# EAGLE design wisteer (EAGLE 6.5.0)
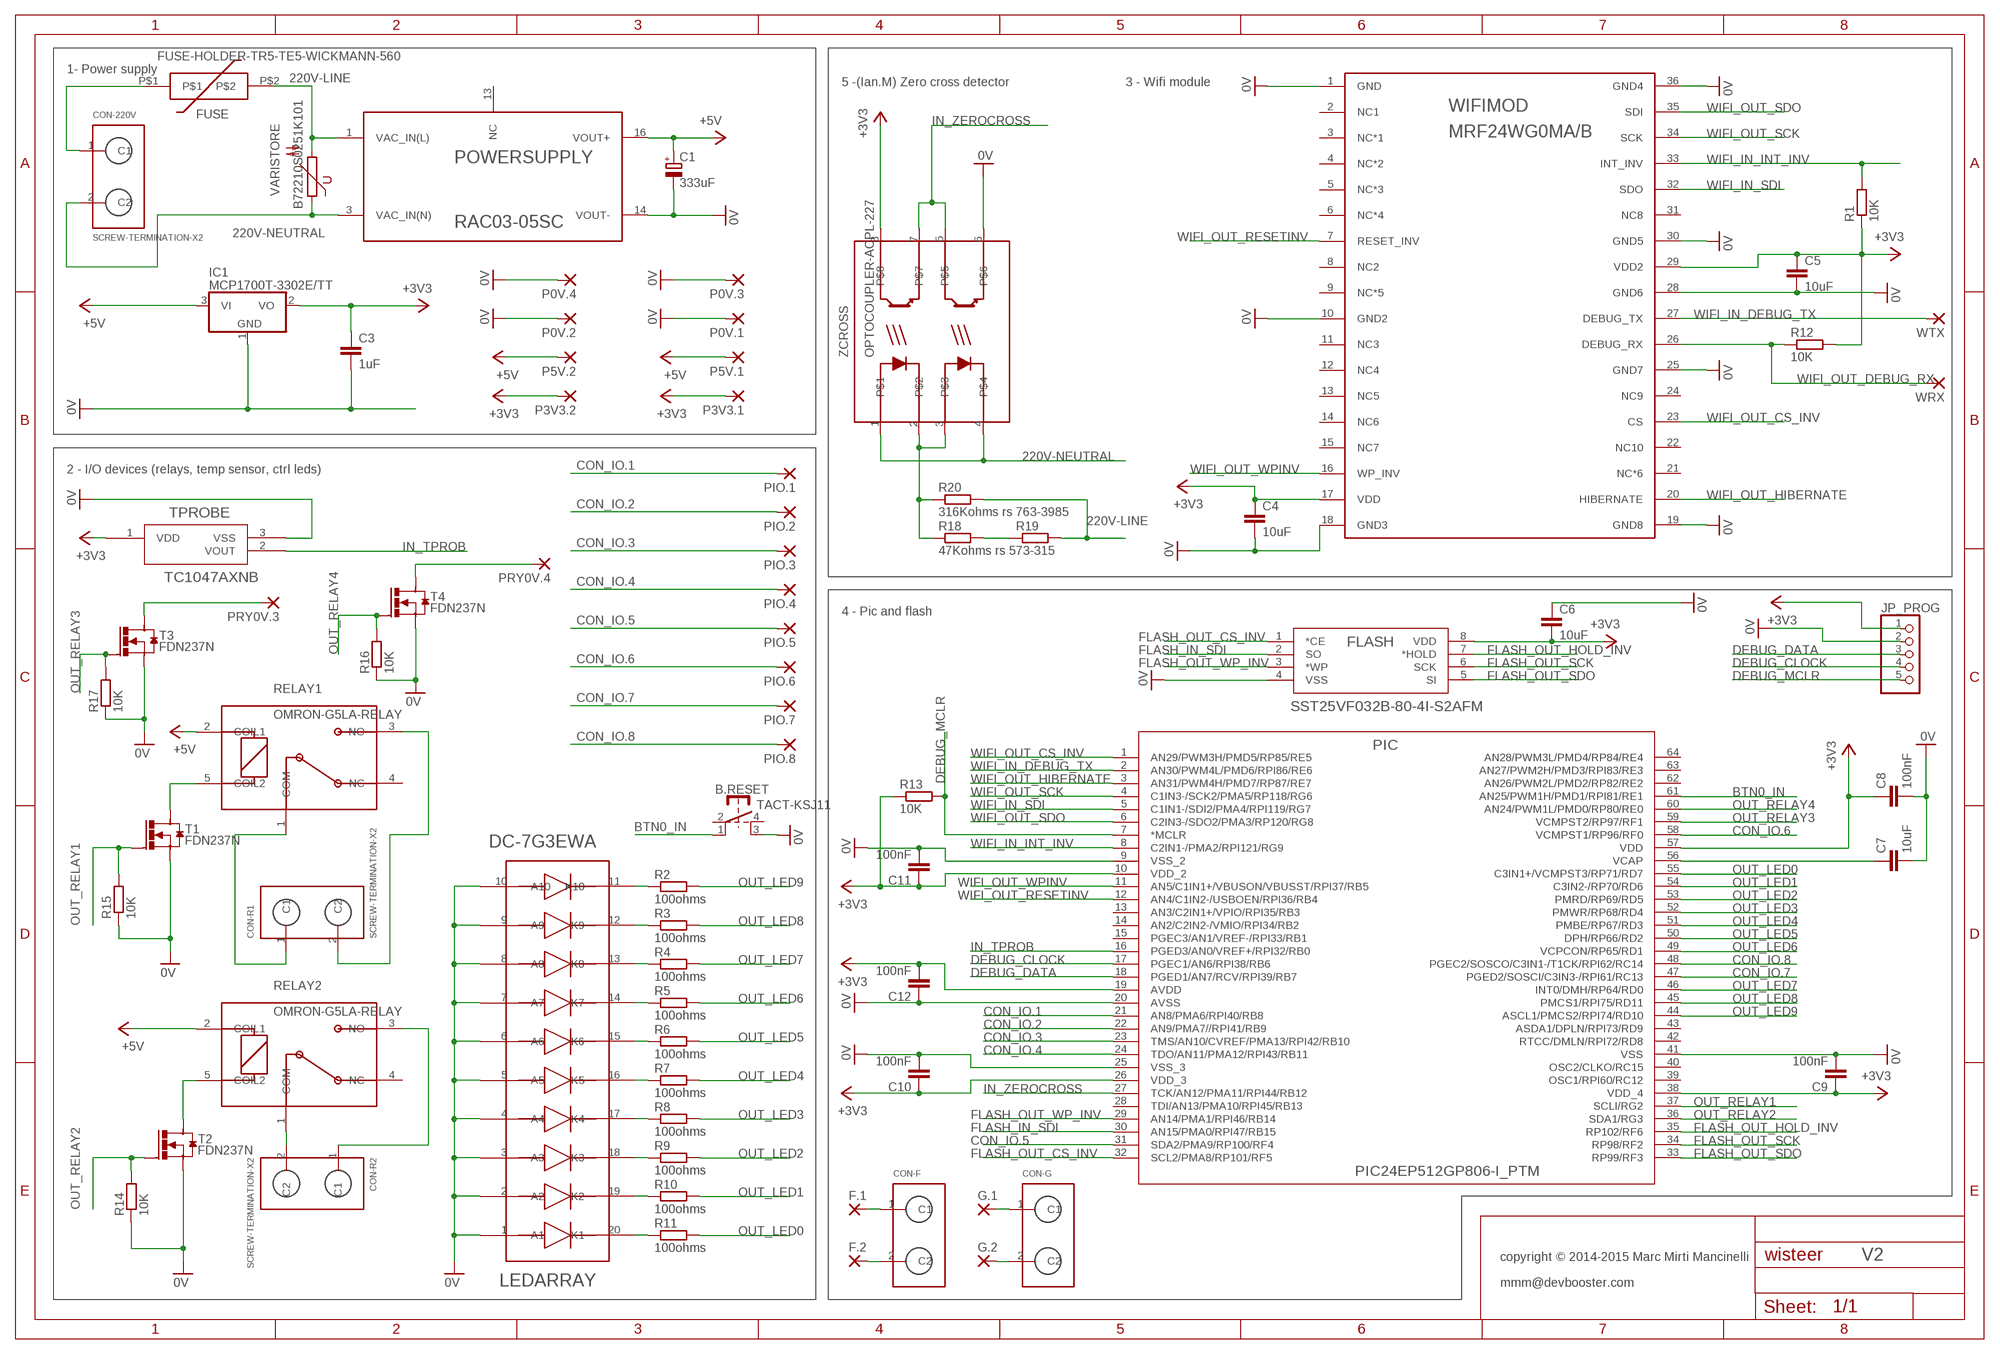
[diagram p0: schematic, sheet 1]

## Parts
B.RESET  TACT-KSJ11  [TACT-KSJ11]
C1  333uF  CPOL-EUTT5D10  [TT5D10]
C3  1uF  C-EUC0805  [C0805]
C4  10uF  C-EUC1210  [C1210]
C5  10uF  C-EUC1210  [C1210]
C6  10uF  C-EUC1210  [C1210]
C7  10uF  C-EUC1210  [C1210]
C8  100nF  C-EUC0603  [C0603]
C9  100nF  C-EUC0603  [C0603]
C10  100nF  C-EUC0603  [C0603]
C11  100nF  C-EUC0603  [C0603]
C12  100nF  C-EUC0603  [C0603]
CON-220V  SCREW-TERMINATION-X2  [PM5.08-2-90]
CON-F  SCREW-TERMINATION-X22.54  [MPT0.5-2-2.54]
CON-G  SCREW-TERMINATION-X22.54  [MPT0.5-2-2.54]
CON-R1  SCREW-TERMINATION-X2  [PM5.08-2-90]
CON-R2  SCREW-TERMINATION-X2  [PM5.08-2-90]
F.1  1,6/0,8  [1,6/0,8]
F.2  1,6/0,8  [1,6/0,8]
FLASH  SST25VF032B-80-4I-S2AFM  [SOIC8_S2A_SST-M]
FUSE  FUSE-HOLDER-TR5-TE5-WICKMANN-560  [FUSE-HOLDER-TR5-TE5-WICKMANN-560]
G.1  1,6/0,8  [1,6/0,8]
G.2  1,6/0,8  [1,6/0,8]
IC1  MCP1700T-3302E/TT  MCP1703CB  [SOT23]
JP_PROG  PINHD-1X5  [1X05]
LEDARRAY  DC-7G3EWA  10-SEGMENT-LED-ARRAY  [10-SEG-LED-DC-7G3EWA]
P0V.1  1,6/0,8  [1,6/0,8]
P0V.2  1,6/0,8  [1,6/0,8]
P0V.3  1,6/0,8  [1,6/0,8]
P0V.4  1,6/0,8  [1,6/0,8]
P3V3.1  1,6/0,8  [1,6/0,8]
P3V3.2  1,6/0,8  [1,6/0,8]
P5V.1  1,6/0,8  [1,6/0,8]
P5V.2  1,6/0,8  [1,6/0,8]
PIC  PIC24EP512GP806-I_PTM  [QFP64-10X10MC-M]
PIO.1  1,6/0,8  [1,6/0,8]
PIO.2  1,6/0,8  [1,6/0,8]
PIO.3  1,6/0,8  [1,6/0,8]
PIO.4  1,6/0,8  [1,6/0,8]
PIO.5  1,6/0,8  [1,6/0,8]
PIO.6  1,6/0,8  [1,6/0,8]
PIO.7  1,6/0,8  [1,6/0,8]
PIO.8  1,6/0,8  [1,6/0,8]
POWERSUPPLY  RAC03-05SC  [RAC03-05SC]
PRY0V.3  1,6/0,8  [1,6/0,8]
PRY0V.4  1,6/0,8  [1,6/0,8]
R1  10K  R-EU_R0603  [R0603]
R2  100ohms  R-EU_R0603  [R0603]
R3  100ohms  R-EU_R0603  [R0603]
R4  100ohms  R-EU_R0603  [R0603]
R5  100ohms  R-EU_R0603  [R0603]
R6  100ohms  R-EU_R0603  [R0603]
R7  100ohms  R-EU_R0603  [R0603]
R8  100ohms  R-EU_R0603  [R0603]
R9  100ohms  R-EU_R0603  [R0603]
R10  100ohms  R-EU_R0603  [R0603]
R11  100ohms  R-EU_R0603  [R0603]
R12  10K  R-EU_R0603  [R0603]
R13  10K  R-EU_R0603  [R0603]
R14  10K  R-EU_R0603  [R0603]
R15  10K  R-EU_R0603  [R0603]
R16  10K  R-EU_R0603  [R0603]
R17  10K  R-EU_R0603  [R0603]
R18  47Kohms rs 573-315  R-EU_R1206W  [R1206W]
R19  47Kohms rs 573-315  R-EU_R1206W  [R1206W]
R20  316Kohms rs 763-3985  R-EU_R0805W  [R0805W]
RELAY1  OMRON-G5LA-RELAY  [OMRON-G5LA-RELAY]
RELAY2  OMRON-G5LA-RELAY  [OMRON-G5LA-RELAY]
T1  FDN237N  [SUPERSOT-3]
T2  FDN237N  [SUPERSOT-3]
T3  FDN237N  [SUPERSOT-3]
T4  FDN237N  [SUPERSOT-3]
TPROBE  TC1047AXNB  [SOT-23_MC]
VARISTORE  B72210S0251K101  S10K250  [S10K250]
WIFIMOD  MRF24WG0MA/B  MRF24WG0MA  [MRF24WG0MA]
WRX  1,6/0,8  [1,6/0,8]
WTX  1,6/0,8  [1,6/0,8]
ZCROSS  OPTOCOUPLER-ACPL-227  [SOIC8_S2A_SST-M]

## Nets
0V: B.RESET.3(S1) C1.- C3.2 C4.2 C5.2 C6.1 C7.2 C8.2 C9.2 C10.2 C11.2 C12.1 FLASH.4(VSS) IC1.1(GND) JP_PROG.2 LEDARRAY.1(A1) LEDARRAY.2(A2) LEDARRAY.3(A3) LEDARRAY.4(A4) LEDARRAY.5(A5) LEDARRAY.6(A6) LEDARRAY.7(A7) LEDARRAY.8(A8) LEDARRAY.9(A9) LEDARRAY.10(A10) P0V.1.1(P) P0V.2.1(P) P0V.3.1(P) P0V.4.1(P) PIC.9(VSS_2) PIC.20(AVSS) PIC.25(VSS_3) PIC.41(VSS) POWERSUPPLY.14(VOUT-) R14.1 R15.1 R16.1 R17.1 T1.2(S) T2.2(S) T3.2(S) T4.2(S) TPROBE.3(VSS) WIFIMOD.1(GND) WIFIMOD.10(GND2) WIFIMOD.18(GND3) WIFIMOD.19(GND8) WIFIMOD.25(GND7) WIFIMOD.28(GND6) WIFIMOD.30(GND5) WIFIMOD.36(GND4) ZCROSS.6
220V-LINE [220VPOWER]: FUSE.P$2 POWERSUPPLY.1(VAC_IN(L)) R19.2 R20.2 VARISTORE.2
220V-NEUTRAL [220VPOWER]: CON-220V.2(C2) POWERSUPPLY.3(VAC_IN(N)) VARISTORE.1 ZCROSS.1 ZCROSS.4
+3V3: C3.1 C4.1 C5.1 C6.2 C8.1 C9.1 C10.1 C11.1 C12.2 FLASH.8(VDD) IC1.2(VO) JP_PROG.1 P3V3.1.1(P) P3V3.2.1(P) PIC.10(VDD_2) PIC.19(AVDD) PIC.26(VDD_3) PIC.38(VDD_4) PIC.57(VDD) R1.1 R12.2 R13.1 TPROBE.1(VDD) WIFIMOD.17(VDD) WIFIMOD.29(VDD2) ZCROSS.8
+5V: C1.+ IC1.3(VI) P5V.1.1(P) P5V.2.1(P) POWERSUPPLY.16(VOUT+) RELAY1.2(COIL1) RELAY2.2(COIL1)
BTN0_IN: B.RESET.1 PIC.61(AN25/PWM1H/PMD1/RPI81/RE1)
CON_IO.1: PIC.21(AN8/PMA6/RPI40/RB8) PIO.1.1(P)
CON_IO.2: PIC.22(AN9/PMA7//RPI41/RB9) PIO.2.1(P)
CON_IO.3: PIC.23(TMS/AN10/CVREF/PMA13/RPI42/RB10) PIO.3.1(P)
CON_IO.4: PIC.24(TDO/AN11/PMA12/RPI43/RB11) PIO.4.1(P)
CON_IO.5: PIC.31(SDA2/PMA9/RP100/RF4) PIO.5.1(P)
CON_IO.6: PIC.58(VCMPST1/RP96/RF0) PIO.6.1(P)
CON_IO.7: PIC.47(PGED2/SOSCI/C3IN3-/RPI61/RC13) PIO.7.1(P)
CON_IO.8: PIC.48(PGEC2/SOSCO/C3IN1-/T1CK/RPI62/RC14) PIO.8.1(P)
DEBUG_CLOCK: JP_PROG.4 PIC.17(PGEC1/AN6/RPI38/RB6)
DEBUG_DATA: JP_PROG.3 PIC.18(PGED1/AN7/RCV/RPI39/RB7)
DEBUG_MCLR: JP_PROG.5 PIC.7(*MCLR) R13.2
FLASH_IN_SDI: FLASH.2(SO) PIC.30(AN15/PMA0/RPI47/RB15)
FLASH_OUT_CS_INV: FLASH.1(*CE) PIC.32(SCL2/PMA8/RP101/RF5)
FLASH_OUT_HOLD_INV: FLASH.7(*HOLD) PIC.35(RP102/RF6)
FLASH_OUT_SCK: FLASH.6(SCK) PIC.34(RP98/RF2)
FLASH_OUT_SDO: FLASH.5(SI) PIC.33(RP99/RF3)
FLASH_OUT_WP_INV: FLASH.3(*WP) PIC.29(AN14/PMA1/RPI46/RB14)
IN_TPROB: PIC.16(PGED3/AN0/VREF+/RPI32/RB0) TPROBE.2(VOUT)
IN_ZEROCROSS: PIC.27(TCK/AN12/PMA11/RPI44/RB12) ZCROSS.5 ZCROSS.7
N$2: R18.1 R20.1 ZCROSS.2 ZCROSS.3
N$3 [220VRELAY]: CON-R2.2(C2) RELAY2.1(COM)
N$4 [220VRELAY]: CON-R2.1(C1) RELAY2.3(NO)
N$5 [220VRELAY]: CON-R1.1(C1) RELAY1.1(COM)
N$6 [220VRELAY]: CON-R1.2(C2) RELAY1.3(NO)
N$7: LEDARRAY.11(K10) R2.1
N$8: RELAY2.5(COIL2) T2.3(D)
N$9: LEDARRAY.12(K9) R3.1
N$10: LEDARRAY.13(K8) R4.1
N$11: LEDARRAY.14(K7) R5.1
N$12: RELAY1.5(COIL2) T1.3(D)
N$13: LEDARRAY.15(K6) R6.1
N$14: LEDARRAY.16(K5) R7.1
N$15: LEDARRAY.17(K4) R8.1
N$16: LEDARRAY.18(K3) R9.1
N$17: LEDARRAY.19(K2) R10.1
N$18: LEDARRAY.20(K1) R11.1
N$19: C7.1 PIC.56(VCAP)
N$20 [220VPOWER]: CON-220V.1(C1) FUSE.P$1
N$21: CON-F.1(C1) F.1.1(P)
N$22: CON-F.2(C2) F.2.1(P)
N$23: CON-G.1(C1) G.1.1(P)
N$24: CON-G.2(C2) G.2.1(P)
N$25: R18.2 R19.1
OUT_LED0: PIC.55(C3IN1+/VCMPST3/RP71/RD7) R11.2
OUT_LED1: PIC.54(C3IN2-/RP70/RD6) R10.2
OUT_LED2: PIC.53(PMRD/RP69/RD5) R9.2
OUT_LED3: PIC.52(PMWR/RP68/RD4) R8.2
OUT_LED4: PIC.51(PMBE/RP67/RD3) R7.2
OUT_LED5: PIC.50(DPH/RP66/RD2) R6.2
OUT_LED6: PIC.49(VCPCON/RP65/RD1) R5.2
OUT_LED7: PIC.46(INT0/DMH/RP64/RD0) R4.2
OUT_LED8: PIC.45(PMCS1/RPI75/RD11) R3.2
OUT_LED9: PIC.44(ASCL1/PMCS2/RPI74/RD10) R2.2
OUT_RELAY1: PIC.37(SCLI/RG2) R15.2 T1.1(G)
OUT_RELAY2: PIC.36(SDA1/RG3) R14.2 T2.1(G)
OUT_RELAY3: PIC.59(VCMPST2/RP97/RF1) R17.2 T3.1(G)
OUT_RELAY4: PIC.60(AN24/PWM1L/PMD0/RP80/RE0) R16.2 T4.1(G)
SRY0V.2: PRY0V.4.1(P) T4.3(D)
SRY0V.3: PRY0V.3.1(P) T3.3(D)
WIFI_IN_DEBUG_TX: PIC.2(AN30/PWM4L/PMD6/RPI86/RE6) WIFIMOD.27(DEBUG_TX) WTX.1(P)
WIFI_IN_INT_INV: PIC.8(C2IN1-/PMA2/RPI121/RG9) R1.2 WIFIMOD.33(INT_INV)
WIFI_IN_SDI: PIC.5(C1IN1-/SDI2/PMA4/RPI119/RG7) WIFIMOD.32(SDO)
WIFI_OUT_CS_INV: PIC.1(AN29/PWM3H/PMD5/RP85/RE5) WIFIMOD.23(CS)
WIFI_OUT_DEBUG_RX: R12.1 WIFIMOD.26(DEBUG_RX) WRX.1(P)
WIFI_OUT_HIBERNATE: PIC.3(AN31/PWM4H/PMD7/RP87/RE7) WIFIMOD.20(HIBERNATE)
WIFI_OUT_RESETINV: PIC.12(AN4/C1IN2-/USBOEN/RPI36/RB4) WIFIMOD.7(RESET_INV)
WIFI_OUT_SCK: PIC.4(C1IN3-/SCK2/PMA5/RP118/RG6) WIFIMOD.34(SCK)
WIFI_OUT_SDO: PIC.6(C2IN3-/SDO2/PMA3/RP120/RG8) WIFIMOD.35(SDI)
WIFI_OUT_WPINV: PIC.11(AN5/C1IN1+/VBUSON/VBUSST/RPI37/RB5) WIFIMOD.16(WP_INV)
Unconnected: B.RESET.2(P) B.RESET.4(S) PIC.13(AN3/C2IN1+/VPIO/RPI35/RB3) PIC.14(AN2/C2IN2-/VMIO/RPI34/RB2) PIC.15(PGEC3/AN1/VREF-/RPI33/RB1) PIC.28(TDI/AN13/PMA10/RPI45/RB13) PIC.39(OSC1/RPI60/RC12) PIC.40(OSC2/CLKO/RC15) PIC.42(RTCC/DMLN/RPI72/RD8) PIC.43(ASDA1/DPLN/RPI73/RD9) PIC.62(AN26/PWM2L/PMD2/RP82/RE2) PIC.63(AN27/PWM2H/PMD3/RPI83/RE3) PIC.64(AN28/PWM3L/PMD4/RP84/RE4) POWERSUPPLY.13(NC) RELAY1.4(NC) RELAY2.4(NC) WIFIMOD.2(NC1) WIFIMOD.3(NC*1) WIFIMOD.4(NC*2) WIFIMOD.5(NC*3) WIFIMOD.6(NC*4) WIFIMOD.8(NC2) WIFIMOD.9(NC*5) WIFIMOD.11(NC3) WIFIMOD.12(NC4) WIFIMOD.13(NC5) WIFIMOD.14(NC6) WIFIMOD.15(NC7) WIFIMOD.21(NC*6) WIFIMOD.22(NC10) WIFIMOD.24(NC9) WIFIMOD.31(NC8)

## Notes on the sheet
- 1- Power supply
- 5 -(Ian.M) Zero cross detector | 3 - Wifi module
- 2 - I/O devices (relays, temp sensor, ctrl leds)
- 4 - Pic and flash
- copyright © 2014-2015 Marc Mirti Mancinelli | V2
- mmm@devbooster.com

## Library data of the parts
B.RESET = mmm:TACT-KSJ11: KSJ11: KSJ Series Spherical Actuator Tact Switches Doc: http://www.madvapes.com/assets/images/ksj11.pdf madvapes ref: Item Id: 10117
C1 = rcl:CPOL-EU: POLARIZED CAPACITOR, European symbol
C3-C12 = rcl:C-EU: CAPACITOR, European symbol
CON-220V CON-F CON-G CON-R1 CON-R2 = comps for wipee:SCREW-TERMINATION-X2: PM5.08-2-90 5.08mm spacement
F.1 F.2 G.1 G.2 P0V.1-P0V.4 P3V3.1 P3V3.2 P5V.1 P5V.2 PIO.1-PIO.8 PRY0V.3 PRY0V.4 WRX WTX = wirepad:1,6/0,8: THROUGH-HOLE PAD
FLASH = comps for wipee:SST25VF032B-80-4I-S2AF: SST25VF032B-50-4I-S2AF: Flash memory (32Mbits) http://ww1.microchip.com/downloads/en/DeviceDoc/25071A.pdf
FUSE = comps for wipee:FUSE-HOLDER-TR5-TE5-WICKMANN-560: TR5/TE5 Fuse
IC1 = linear:MCP1703: 250 mA, 16V, Low Quiescent Current LDO Regulator Source: http://ww1.microchip.com/downloads/en/DeviceDoc/22049b.pdf
JP_PROG = pinhead:PINHD-1X5: PIN HEADER
LEDARRAY = comps for wipee:10-SEGMENT-LED-ARRAY: DC-7G3EWA :led array (rs 247-3107) http://radiospares-fr.rs-online.com/web/p/afficheurs-led/2473107/
PIC = comps for wipee:PIC24EP512GP806-I_PT: PIC24EP512GP806-I/PT: Pic with 512KB rom, 50KB ram, 60/70Mhz, 64 pins http://ww1.microchip.com/downloads/en/DeviceDoc/70616g.pdf
POWERSUPPLY = comps for wipee:RAC03-05SC: RAC03-05SC Power supply http://radiospares-fr.rs-online.com/web/p/alimentations-a-decoupage-integrables/7398339/
R1-R20 = rcl:R-EU_: RESISTOR, European symbol
RELAY1 RELAY2 = comps for wipee:OMRON-G5LA-RELAY: OMRON-G5LA-RELAY 5v, SPDT, 0.36W http://radiospares-fr.rs-online.com/web/p/relais-sans-accrochage/6839138/
T1-T4 = mmm:FDN237N: MOSFET CANAL N FDN237N Fairchild semiconductors http://docs-europe.electrocomponents.com/webdocs/0d23/0900766b80d23106.pdf
TPROBE = microchip tfrog:TC1047AXNB: Temperature sensor (TC1047AVNBTR) TC1047A can accurately measure temperature from -40C to +125C. For the TC1047A, the output voltage range is typically 100mV at -40C, 500mV at 0C, 750mV at +25C, and 1.75V at +125C. A 10mV/°C http://www.microchip.com/wwwproducts/Devices.aspx?dDocName=en010753#1
VARISTORE = varistor:S10K250: VARISTOR
WIFIMOD = comps for wipee:MRF24WG0MA: MRF24WG0MA Wifi module G/B with integrated antenna. http://ww1.microchip.com/downloads/en/DeviceDoc/70686B.pdf
ZCROSS = comps for wipee:OPTOCOUPLER-ACPL-227: Avago ACPL-227-50CE DC Input, Transistor Output Dual Optocoupler, SMT SOIC 8 2 channels, 50ma, 1.4v, delays 2us-3us Doc: http://docs-europe.electrocomponents.com/webdocs/0db7/0900766b80db7ce4.pdf Ref RS: 693-6797

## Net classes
0 default: clearance 0.205 mm
1 220VPOWER: clearance 0.5 mm
2 220VRELAY: clearance 0.5 mm

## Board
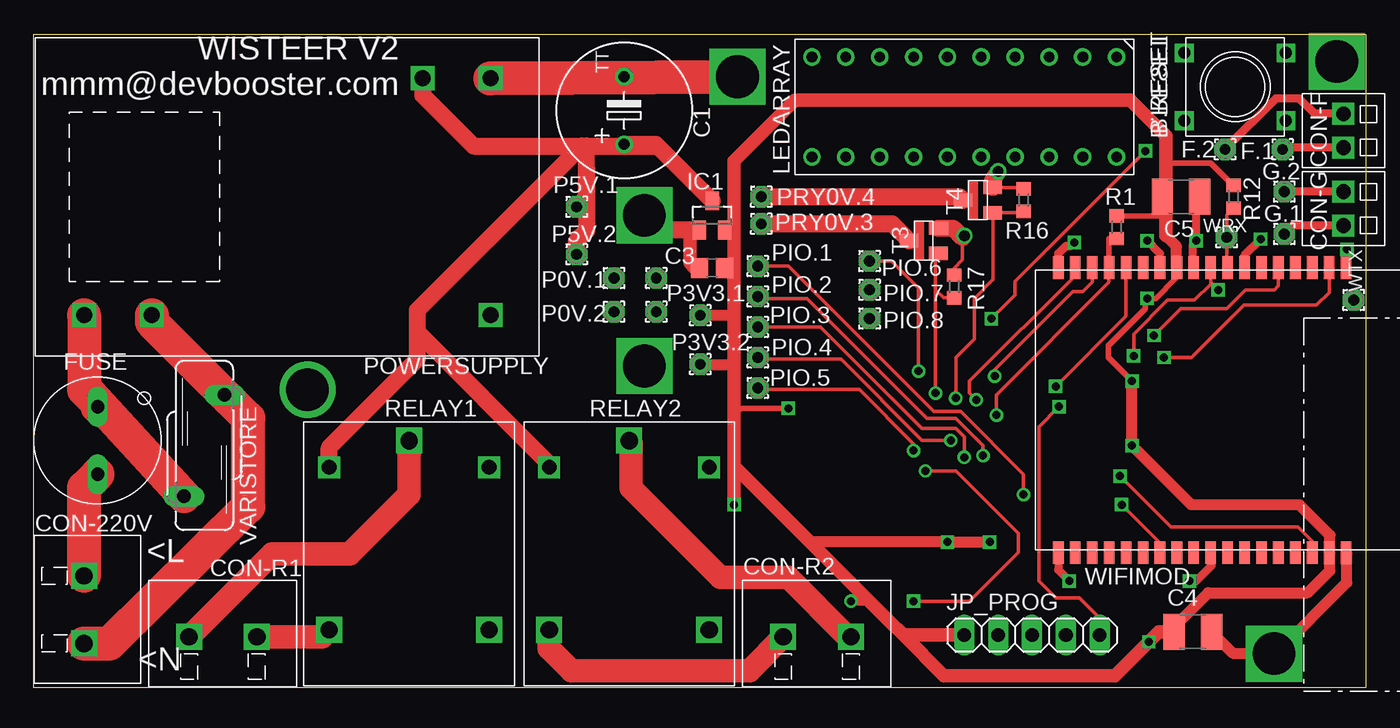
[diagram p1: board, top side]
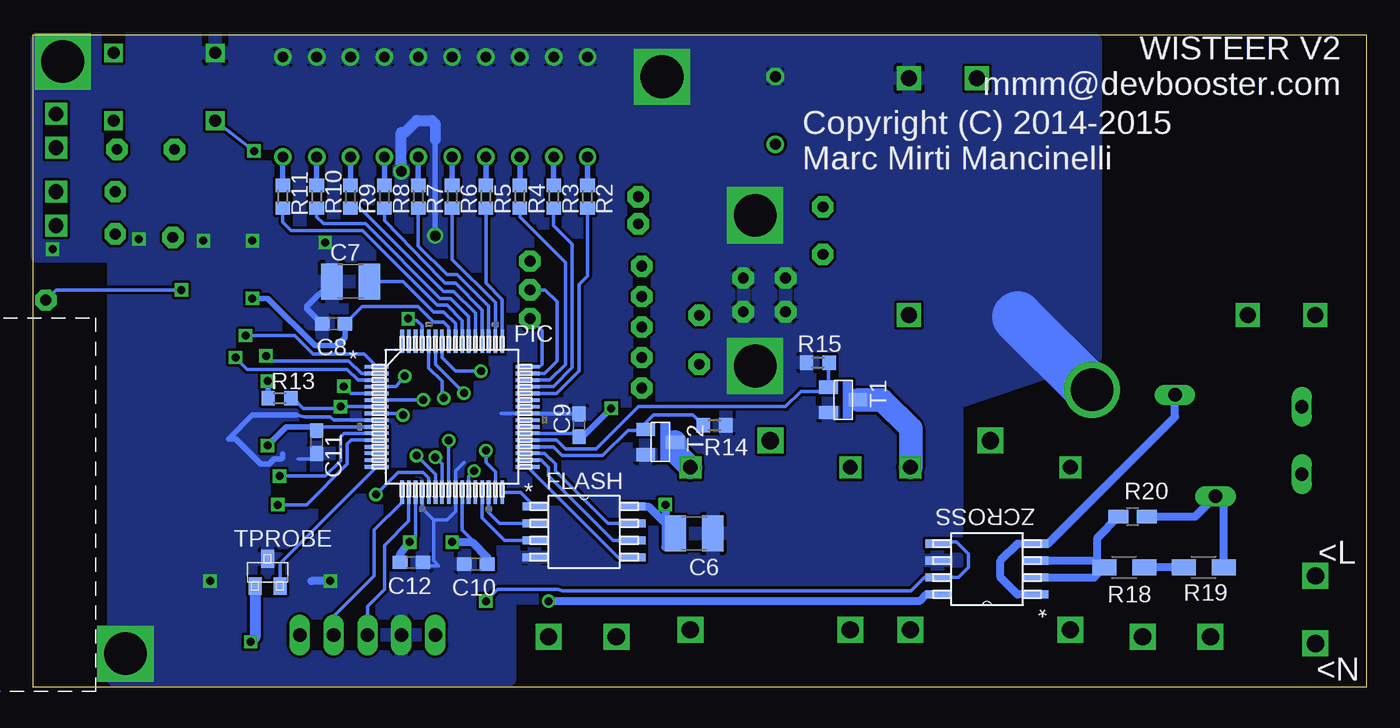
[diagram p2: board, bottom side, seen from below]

Size 100 x 49 mm. Coordinates in mm from the lower left corner, seen from the top.
Outline: 0,0 100,0 100,49 0,49 0,0
Copper layers (1*16): Top 0.035mm / dielectric 1.5mm / Bottom 0.035mm
Design rules "default *": minimum track width 10mil, minimum drill 16mil, track to track 8mil, track to pad 8mil, pad to pad 8mil, via to via 8mil, smd to smd 8mil, copper to edge 0mil, drill to drill 8mil, minimum pad ring 10mil, minimum via ring 8mil, stop-mask expansion 4mil, vias tented up to drill 0mil, thermal gap 10mil

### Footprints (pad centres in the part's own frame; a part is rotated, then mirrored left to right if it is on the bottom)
TACT-KSJ11 = drill 0.9 square: 1 -3.81,-2.54; 2 3.81,-2.54; 3 -3.81,2.54; 4 3.81,2.54
TT5D10 = drill 0.813: + -2.54,0 | drill 0.813 octagon: - 2.54,0
C0805 = smd 1.3 x 1.5: 1 -0.95,0; 2 0.95,0
C1210 = smd 1.6 x 2.7: 1 -1.4,0; 2 1.4,0
C0603 = smd 1.1 x 1: 1 -0.85,0; 2 0.85,0
PM5.08-2-90 = drill 1.3 square: 1 -2.54,0; 2 2.54,0
MPT0.5-2-2.54 = drill 1.1 square: 1 -1.27,0; 2 1.27,0
1,6/0,8 = drill 0.813 pad 1.6 octagon: 1 0,0
SOIC8_S2A_SST-M = smd 1.829 x 0.61: 1 -3.708,1.905; 2 -3.708,0.635; 3 -3.708,-0.635; 4 -3.708,-1.905; 5 3.708,-1.905; 6 3.708,-0.635; 7 3.708,0.635; 8 3.708,1.905
FUSE-HOLDER-TR5-TE5-WICKMANN-560 = drill 1 long: P$1 -2.54,0; P$2 2.54,0
SOT23 = smd 1 x 1.4: 1 -0.95,-1.1; 2 0.95,-1.1; 3 0,1.1
1X05 = drill 1.016 long: 1 -5.08,0; 2 -2.54,0; 3 0,0; 4 2.54,0; 5 5.08,0
10-SEG-LED-DC-7G3EWA = drill 0.8: 1 -11.43,-3.75; 2 -8.89,-3.75; 3 -6.35,-3.75; 4 -3.81,-3.75; 5 -1.27,-3.75; 6 1.27,-3.75; 7 3.81,-3.75; 8 6.35,-3.75; 9 8.89,-3.75; 10 11.43,-3.75; 11 11.43,3.75; 12 8.89,3.75; 13 6.35,3.75; 14 3.81,3.75; 15 1.27,3.75; 16 -1.27,3.75; 17 -3.81,3.75; 18 -6.35,3.75; 19 -8.89,3.75; 20 -11.43,3.75
QFP64-10X10MC-M = smd 1.778 x 0.279: 1 -5.664,3.759; 2 -5.664,3.251; 3 -5.664,2.743; 4 -5.664,2.261; 5 -5.664,1.753; 6 -5.664,1.245; 7 -5.664,0.762; 8 -5.664,0.254; 9 -5.664,-0.254; 10 -5.664,-0.762; 11 -5.664,-1.245; 12 -5.664,-1.753; 13 -5.664,-2.261; 14 -5.664,-2.743; 15 -5.664,-3.251; 16 -5.664,-3.759; 33 5.664,-3.759; 34 5.664,-3.251; 35 5.664,-2.743; 36 5.664,-2.261; 37 5.664,-1.753; 38 5.664,-1.245; 39 5.664,-0.762; 40 5.664,-0.254; 41 5.664,0.254; 42 5.664,0.762; 43 5.664,1.245; 44 5.664,1.753; 45 5.664,2.261; 46 5.664,2.743; 47 5.664,3.251; 48 5.664,3.759 | smd 0.279 x 1.778: 17 -3.759,-5.664; 18 -3.251,-5.664; 19 -2.743,-5.664; 20 -2.261,-5.664; 21 -1.753,-5.664; 22 -1.245,-5.664; 23 -0.762,-5.664; 24 -0.254,-5.664; 25 0.254,-5.664; 26 0.762,-5.664; 27 1.245,-5.664; 28 1.753,-5.664; 29 2.261,-5.664; 30 2.743,-5.664; 31 3.251,-5.664; 32 3.759,-5.664; 49 3.759,5.664; 50 3.251,5.664; 51 2.743,5.664; 52 2.261,5.664; 53 1.753,5.664; 54 1.245,5.664; 55 0.762,5.664; 56 0.254,5.664; 57 -0.254,5.664; 58 -0.762,5.664; 59 -1.245,5.664; 60 -1.753,5.664; 61 -2.261,5.664; 62 -2.743,5.664; 63 -3.251,5.664; 64 -3.759,5.664
RAC03-05SC = drill 1.2 square: 1 -15.24,-8.89; 3 -10.16,-8.89; 13 15.24,-8.89; 14 15.24,8.89; 16 10.16,8.89
R0603 = smd 1 x 1.1: 1 -0.85,0; 2 0.85,0
R1206W = smd 1.8 x 1.2: 1 -1.499,0; 2 1.499,0
R0805W = smd 1.5 x 1: 1 -1.052,0; 2 1.052,0
OMRON-G5LA-RELAY = drill 1.3 square: 1 -8.5,0; 3 5.7,-6; 4 5.7,6 | drill 1.1 square: 2 -6.5,-6; 5 -6.5,6
SUPERSOT-3 = smd 1 x 1.4: 1 -0.95,-1.1; 2 0.95,-1.1; 3 0,1.1
SOT-23_MC = smd 0.991 x 1.321: 1 -0.94,-1.016; 2 0.94,-1.016; 3 0,1.016
S10K250 = drill 1.016 long: 1 -1.524,-3.81; 2 1.524,3.81
MRF24WG0MA = smd 1.7 x 0.8: 1 -10.2,13.27; 2 -10.2,12; 3 -10.2,10.73; 4 -10.2,9.46; 5 -10.2,8.19; 6 -10.2,6.92; 7 -10.2,5.65; 8 -10.2,4.38; 9 -10.2,3.11; 10 -10.2,1.84; 11 -10.2,0.57; 12 -10.2,-0.7; 13 -10.2,-1.97; 14 -10.2,-3.24; 15 -10.2,-4.51; 16 -10.2,-5.78; 17 -10.2,-7.05; 18 -10.2,-8.32; 19 11.2,-8.32; 20 11.2,-7.05; 21 11.2,-5.78; 22 11.2,-4.51; 23 11.2,-3.24; 24 11.2,-1.97; 25 11.2,-0.7; 26 11.2,0.57; 27 11.2,1.84; 28 11.2,3.11; 29 11.2,4.38; 30 11.2,5.65; 31 11.2,6.92; 32 11.2,8.19; 33 11.2,9.46; 34 11.2,10.73; 35 11.2,12; 36 11.2,13.27

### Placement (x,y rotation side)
B.RESET  90.17,45.09 0 top
C1  44.32,43.31 90 top
C3  50.93,31.5 180 top
C4  87,4.19 0 top
C5  86.11,36.83 0 top
C6  50.42,11.56 180 bottom
C7  76.2,30.48 180 bottom
C8  77.47,27.3 180 bottom
C9  59.05,19.68 90 bottom
C10  66.8,9.27 180 bottom
C11  78.74,18.41 270 bottom
C12  71.63,9.4 180 bottom
CON-220V  3.81,5.84 270 top
CON-F  98.3,41.78 90 top
CON-G  98.3,35.94 90 top
CON-R1  14.22,3.81 0 top
CON-R2  58.8,3.81 0 top
F.1  93.73,40.39 0 top
F.2  89.41,40.39 0 top
FLASH  58.67,11.68 0 bottom
FUSE  4.83,18.54 90 top
G.1  93.85,34.04 0 top
G.2  93.85,37.21 0 top
IC1  50.93,35.43 0 top
JP_PROG  74.93,3.94 0 top
LEDARRAY  69.85,43.56 180 top
P0V.1  43.56,30.73 0 top
P0V.2  43.56,28.19 0 top
P0V.3  46.74,30.73 0 top
P0V.4  46.74,28.19 0 top
P3V3.1  50.04,27.94 0 top
P3V3.2  50.04,24.26 0 top
P5V.1  40.77,36.07 0 top
P5V.2  40.77,32.51 0 top
PIC  68.58,20.32 0 bottom
PIO.1  54.36,31.62 0 top
PIO.2  54.36,29.34 0 top
PIO.3  54.36,27.05 0 top
PIO.4  54.36,24.77 0 top
PIO.5  54.36,22.48 0 top
PIO.6  62.74,32 0 top
PIO.7  62.74,29.84 0 top
PIO.8  62.74,27.69 0 top
POWERSUPPLY  19.05,36.83 0 top
PRY0V.3  54.61,34.8 0 top
PRY0V.4  54.61,36.83 0 top
R1  81.28,34.54 270 top
R2  58.42,36.83 270 bottom
R3  60.96,36.83 270 bottom
R4  63.5,36.83 270 bottom
R5  66.04,36.83 270 bottom
R6  68.58,36.83 270 bottom
R7  71.12,36.83 270 bottom
R8  73.66,36.83 270 bottom
R9  76.2,36.83 270 bottom
R10  78.74,36.83 270 bottom
R11  81.28,36.83 270 bottom
R12  90.04,36.83 90 top
R13  81.53,21.72 0 bottom
R14  48.9,19.68 180 bottom
R15  41.15,24.38 0 bottom
R16  74.3,36.58 270 top
R17  69.09,30.1 270 top
R18  18.16,9.02 0 bottom
R19  12.19,9.02 0 bottom
R20  17.53,12.83 0 bottom
RELAY1  28.19,10.03 270 top
RELAY2  44.7,10.03 270 top
T1  39.24,21.59 270 bottom
T2  52.96,18.41 270 bottom
T3  66.8,33.53 90 top
T4  70.87,36.58 90 top
TPROBE  82.42,8.64 0 bottom
VARISTORE  12.83,18.16 180 top
WIFIMOD  90.17,20.32 90 top
WRX  89.53,33.78 0 top
WTX  99.06,29.08 0 top
ZCROSS  28.45,8.89 180 bottom

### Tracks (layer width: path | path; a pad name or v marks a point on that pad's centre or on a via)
0V  (via drill 0.6, 0.8, 3.2)
  Top 0.254: R17.1 69.09,31.5 69.72,32.13 69.72,33.78 | T4.2 74.19,37.53 R16.1
  Top 0.406: 87,31.59 WIFIMOD.28
  Top 0.61: v86.74,8 87.25,8 88.39,9.14 88.39,10.06 WIFIMOD.10 | WIFIMOD.1 76.9,8.82 v77.72,8 | WIFIMOD.30 84.52,32.57 v83.57,33.53 | WIFIMOD.36 76.9,32.58 77.47,33.15 77.85,33.15 v78.11,33.4 | WIFIMOD.19 98.49,32.32 v98.55,32.89 | WIFIMOD.25 90.87,32.45 v92.08,33.66 | 87,31.59 87,33.27 v87.25,33.53 87.25,36.57 C5.2
  Top 0.813: WIFIMOD.18 98.55,10.06 98.55,7.87 93.22,2.54 v93.09,2.54 90.05,2.54 C4.2 | 69.72,33.78 v69.85,33.91
  Top 1.016: C3.2 49.66,31.5 49.28,31.88 49.28,34.21 49.4,34.33 IC1.1
  Top 1.27: 49.4,34.33 46.95,34.33 v45.85,35.43 | T4.2 71.97,38.06 v72.39,38.73 | T3.2 69.03,34.48 69.72,33.78
  Top 2.54: POWERSUPPLY.14 v52.83,45.85
  Bottom 0.254: PIC.9 77.47,20.07 77.72,20.32 79.63,20.32 80.26,20.45 | 80.14,17.14 79.16,17.14 C11.2 | PIC.41 64.9,20.57 | 67.69,16.89 68.33,16.26 PIC.25 68.33,13.21 68.96,12.57 69.98,12.57 | PIC.20 70.84,13.44 69.98,12.57 | 69.98,12.57 69.98,9.53 69.6,9.14 70.52,9.14 C12.1
  Bottom 0.305: PIC.41 59.09,20.57 C9.2
  Bottom 0.406: C8.2 78.36,27.3 79.5,28.45 79.5,28.58 C7.2 | 80.26,20.45 83.57,20.45 85.34,18.67 84.84,18.67 82.93,16.76 82.3,16.76 81.92,17.14 81.41,17.14 81.28,17.27 81.28,17.53 | v69.85,33.91 69.85,41.15
  Bottom 0.61: v77.72,8 79.12,8
  Bottom 0.813: v72.39,38.73 72.39,41.66 72.14,41.66 71.25,42.55 70.1,42.55 69.85,42.29 69.85,41.15
  Bottom 3.81: v20.57,22.35 20.7,22.35 26.16,27.81
  other vias: 97.79,46.99 45.85,24.13
  pour Bottom: 30.73,6.73 30.73,21.34 20.32,24.89 20.32,48.53 99.69,48.53 99.69,32.38 93.98,32.38 93.98,0.64 64.26,0.64 64.26,6.73
220V-LINE
  Top 2.54: POWERSUPPLY.1 3.81,22.35 | VARISTORE.2 4.19,22.1 3.81,22.35 | 3.81,22.35 5.33,20.83 5.08,20.83 FUSE.P$2
  Bottom 0.61: R20.2 12.83,12.83 VARISTORE.2 10.69,13.74 R19.2
220V-NEUTRAL
  Top 2.54: CON-220V.2 5.71,3.3 16.13,13.59 16.13,20.19 VARISTORE.1 8.89,27.43 POWERSUPPLY.3
  Bottom 0.61: ZCROSS.1 26.16,6.99 27.43,8.26 27.43,9.53 26.16,10.79 ZCROSS.4 23.88,10.79 14.35,20.32 VARISTORE.1
+3V3  (via drill 0.6)
  Top 0.305: WIFIMOD.29 85.79,33.08
  Top 0.406: 85.72,33.02 84.96,33.78 C5.1 85.09,36.96 85.09,39.37 88.35,39.37 R12.2 | 85.72,31.59 WIFIMOD.29 85.72,31.45 85.72,30.73 84.2,29.21 v83.57,29.21 83.44,29.08 83.44,28.45 80.64,25.65 80.64,24.77 v82.42,22.99 | v56.64,20.95 53.09,20.95 52.58,20.45 | R1.1 84.96,35.39 84.96,36.32
  Top 0.61: 85.59,4.57 C4.1 | 97.28,10.06 WIFIMOD.17 | v61.34,6.48 62.61,6.48 62.67,6.54
  Top 0.813: 85.72,33.02 85.72,31.59 | 85.59,4.57 88.14,7.11 95.63,7.11 97.28,8.76 97.28,10.06 | 85.79,33.08 84.96,33.91 | v82.42,22.99 v82.42,18.16 86.87,13.72 95,13.72 97.28,11.43 97.28,10.54 | P3V3.2.1 52.32,24.26 52.58,24.51 | P3V3.1.1 52.45,27.94 52.58,28.07 | v71.75,10.92 v68.58,10.92 58.36,10.92 58.36,10.86 | 64.9,4.32 64.39,4.83
  Top 1.016: C4.1 84.45,4.19 v83.69,3.43 81.15,0.89 68.33,0.89 65.28,3.94 | v52.58,13.72 52.58,16.64 | 52.58,16.64 52.58,20.45 52.58,24.51 52.58,28.07 52.58,31.5 | 84.96,33.91 84.96,36.32 84.96,41.4 82.3,44.07 57.15,44.07 52.58,39.5 52.58,34.67 | 64.64,4.57 64.39,4.83 62.67,6.54 58.36,10.86 52.58,16.64 | 52.58,31.5 52.58,34.67 | IC1.2 52.24,34.33 52.58,34.67 | C3.1 52.58,31.5 | 64.9,4.32 65.28,3.94 | 65.28,3.94 JP_PROG.1
  Bottom 0.254: PIC.19 71.32,11.35 v71.75,10.92 72.48,10.2 72.48,9.91 C12.2 72.52,9.44 | PIC.10 78.45,19.56 | 78.45,19.56 C11.1 | 78.45,19.56 79.25,19.56 | PIC.57 68.83,27.05 69.22,27.43 69.98,27.43 71.12,28.57 75.35,28.57 C8.1 | PIC.38 59.3,19.07 C9.1 | PIC.26 67.82,11.81 65.95,9.95 65.95,9.78 C10.1
  Bottom 0.406: C9.1 58.76,18.84 v56.64,20.95 | C8.1 76.62,26.25 77.22,25.65 78.87,25.65 82.42,29.21 v83.57,29.21 | R13.1 82.38,22.82 v82.42,22.99 | 79.25,19.56 81.03,19.56 v82.42,18.16
  Bottom 0.61: 83.49,3.63 v83.69,3.43 | v52.58,13.72 52.58,10.54 C6.2 53.85,13.59 FLASH.8 | v71.75,10.92 72.52,9.95 72.48,9.91 | v68.58,10.92 67.09,10.92 65.95,9.78 | ZCROSS.8 33.02,6.99 33.53,6.48 v61.34,6.48
  Bottom 0.813: TPROBE.1 83.36,3.76 v83.69,3.43
+5V
  Top 1.27: POWERSUPPLY.16 29.21,44.45 33.02,40.64 41.15,40.64 | 41.15,40.64 41.48,40.64 | 41.48,40.64 41.48,38.99 | 41.48,38.99 41.48,36.78 P5V.1.1 | P5V.2.1 40.77,33.53 41.53,34.29 41.53,38.94 41.48,38.99 | RELAY1.2 22.19,18 28.83,24.64 28.83,26.67 | 28.83,26.67 28.83,28.32 41.15,40.64 | RELAY2.2 38.7,16.8 28.83,26.67 | 41.48,40.64 46.82,40.64 IC1.3 46.69,40.77 C1.+
BTN0_IN  (via drill 0.6)
  Top 0.254: v83.44,40.26 73.66,30.48 73.66,29.46 v71.88,27.69
  Bottom 0.254: v71.88,27.69 71.75,27.56 71.25,27.56 70.84,27.15 PIC.61 | v83.44,40.26 B.RESET.1
CON_IO.1  (via drill 0.6)
  Top 0.254: v74.3,14.48 74.3,16 69.6,20.7 67.56,20.7 56.64,31.62 PIO.1.1
  Bottom 0.254: PIC.21 70.33,15.72 70.74,16.13 72.64,16.13 v74.3,14.48
CON_IO.2  (via drill 0.6)
  Top 0.254: v71.25,17.4 71.25,18.16 69.22,20.19 67.06,20.19 58.04,29.21 54.48,29.21 PIO.2.1
  Bottom 0.254: PIC.22 69.83,15.98 v71.25,17.4
CON_IO.3  (via drill 0.6)
  Top 0.254: v69.85,17.27 69.85,18.8 69.22,19.43 66.67,19.43 59.05,27.05 PIO.3.1
  Bottom 0.254: PIC.23 69.34,16.76 v69.85,17.27
CON_IO.4  (via drill 0.6)
  Top 0.254: v68.83,18.54 66.67,18.54 60.58,24.64 54.48,24.64 PIO.4.1
  Bottom 0.254: PIC.24 v68.83,18.54
CON_IO.5  (via drill 0.6)
  Top 0.254: PIO.5.1 54.48,22.35 61.98,22.35 66.04,18.29 v66.04,17.78
  Bottom 0.254: PIC.31 65.33,16.18 66.04,16.89 v66.04,17.78
CON_IO.6  (via drill 0.6)
  Top 0.254: v66.42,23.75 66.42,29.97 64.39,32 PIO.6.1
  Bottom 0.254: PIC.58 69.34,24.77 68.33,23.75 v66.42,23.75
CON_IO.7
  Bottom 0.254: PIO.7.1 61.59,29.84 60.71,28.96 60.71,24.51 61.65,23.57 PIC.47
CON_IO.8
  Bottom 0.254: PIC.48 62.03,24.08 61.85,24.26 61.85,26.8 PIO.8.1
DEBUG_CLOCK
  Bottom 0.254: PIC.17 72.34,13.89 74.42,11.81 74.42,8.38 77.47,5.33 JP_PROG.4
DEBUG_DATA
  Bottom 0.254: PIC.18 71.83,12.5 73.66,10.67 73.66,7.37 74.93,6.1 JP_PROG.3
DEBUG_MCLR  (via drill 0.6)
  Top 0.254: v76.96,21.08 75.44,19.56 75.44,8 76.71,6.73 78.49,6.73 79.88,5.33 79.88,4.06 JP_PROG.5
  Bottom 0.254: PIC.7 v76.96,21.08 77.09,20.95 79.76,20.95 80.52,21.72 R13.2
FLASH_IN_SDI
  Bottom 0.254: PIC.30 65.84,13.13 65.02,12.32 FLASH.2
FLASH_OUT_CS_INV
  Bottom 0.254: PIC.32 63.45,14.66 FLASH.1
FLASH_OUT_HOLD_INV
  Bottom 0.254: PIC.35 61.65,17.58 60.83,16.76 60.83,16.26 56.9,12.32 FLASH.7
FLASH_OUT_SCK
  Bottom 0.254: PIC.34 61.9,17.07 61.34,16.51 61.34,15.88 56.52,11.05 FLASH.6
FLASH_OUT_SDO
  Bottom 0.254: PIC.33 56.13,9.78 FLASH.5
FLASH_OUT_WP_INV
  Bottom 0.254: PIC.29 66.32,12.72 64.64,11.05 FLASH.3
IN_TPROB
  Bottom 0.254: TPROBE.2 81.48,9.32 PIC.16
IN_ZEROCROSS  (via drill 0.6)
  Top 0.254: v66.04,6.48 70.23,6.48 73.91,10.16 73.91,11.56 69.22,16.26 v66.93,16.26
  Bottom 0.254: ZCROSS.5 32.03,10.92 30.73,10.92 29.84,10.03 29.84,9.02 30.61,8.26 ZCROSS.7 33.15,8.26 34.16,7.24 60.33,7.24 60.58,7.37 65.15,7.37 v66.04,6.48 | PIC.27 67.33,15.85 v66.93,16.26
N$2
  Bottom 0.61: 23.11,8.26 ZCROSS.2 20.42,8.26 R18.1 20.17,9.53 | ZCROSS.3 20.17,9.53 | 20.17,9.53 20.17,11.24 R20.1
N$3
  Top 1.778: CON-R2.2 61.09,3.81 56.64,8.26 51.56,8.26 44.83,14.99 44.83,18.41 RELAY2.1
N$4
  Top 1.778: RELAY2.3 38.7,2.95 40.39,1.27 53.72,1.27 CON-R2.1
N$5
  Top 1.778: RELAY1.1 28.19,14.48 23.75,10.03 17.91,10.03 CON-R1.1
N$6
  Top 1.778: CON-R1.2 21.67,3.81 RELAY1.3
N$7
  Bottom 0.406: LEDARRAY.11 R2.1
N$8
  Bottom 1.778: 50.73,16.51 RELAY2.5 51.86,17.69 T2.3
N$9
  Bottom 0.406: LEDARRAY.12 R3.1
N$10
  Bottom 0.406: R4.1 LEDARRAY.13
N$11
  Bottom 0.406: LEDARRAY.14 R5.1
N$12
  Bottom 1.778: T1.3 36.32,21.59 34.16,19.43 34.16,16.56 RELAY1.5
N$13
  Bottom 0.406: LEDARRAY.15 R6.1
N$14
  Bottom 0.406: LEDARRAY.16 R7.1
N$15
  Bottom 0.406: LEDARRAY.17 R8.1
N$16
  Bottom 0.406: LEDARRAY.18 R9.1
N$17
  Bottom 0.406: LEDARRAY.19 R10.1
N$18
  Bottom 0.406: LEDARRAY.20 R11.1
N$19
  Bottom 0.254: C7.1 72.26,30.48 69.98,28.19 69.22,28.19 68.33,27.3 PIC.56
N$20
  Top 2.54: CON-220V.1 3.81,14.99 FUSE.P$1
N$21
  Top 0.61: CON-F.1 93.85,40.51 F.1.1
N$22
  Top 0.61: CON-F.2 96.14,43.05 95,44.2 93.22,44.2 F.2.1
N$23
  Top 0.61: CON-G.1 94.49,34.67 G.1.1
N$24
  Top 0.61: CON-G.2 G.2.1
N$25
  Bottom 0.61: R19.1 R18.2
OUT_LED0
  Bottom 0.254: R11.2 81.28,34.92 80.64,34.29 75.31,34.29 69.72,28.7 68.96,28.7 67.82,27.56 PIC.55
OUT_LED1
  Bottom 0.254: R10.2 78.74,35.31 78.23,34.8 75.06,34.8 69.47,29.21 68.71,29.21 67.33,27.84 PIC.54
OUT_LED2
  Bottom 0.254: R9.2 75.48,35.98 69.22,29.72 68.45,29.72 66.83,28.09 | 66.83,28.09 66.8,28.07 | PIC.53 66.83,28.09
OUT_LED3
  Bottom 0.254: R8.2 73.66,35.05 69.47,30.73 69.09,30.35 68.33,30.35 66.32,28.35 PIC.52
OUT_LED4
  Bottom 0.254: R7.2 71.12,33.15 68.96,30.99 68.2,30.99 65.84,28.63 PIC.51
OUT_LED5
  Bottom 0.254: R6.2 68.58,32.13 65.33,28.88 PIC.50
OUT_LED6
  Bottom 0.254: R5.2 66.04,30.35 64.82,29.13 PIC.49
OUT_LED7
  Bottom 0.254: R4.2 63.5,35.31 60.07,31.88 60.07,24.26 61.27,23.06 PIC.46
OUT_LED8
  Bottom 0.254: R3.2 60.96,34.67 59.56,33.27 59.56,24 60.98,22.58 PIC.45
OUT_LED9
  Bottom 0.254: R2.2 58.42,30.86 59.05,30.23 59.05,23.75 60.73,22.07 PIC.44
OUT_RELAY1
  Bottom 0.254: PIC.37 60.73,18.57 60.07,17.91 57.78,17.91 54.61,21.08 43.56,21.08 42.42,22.23 40.66,22.23 T1.1 40.34,24.38
  Bottom 0.406: R15.2 40.34,24.38
OUT_RELAY2
  Bottom 0.254: PIC.36 60.98,18.06 60.33,17.4 57.28,17.4 55.37,19.3 54.12,19.3 T2.1 54.06,19.86 53.47,20.45 50.51,20.45 R14.2
OUT_RELAY3  (via drill 0.6)
  Top 0.254: v67.69,22.1 67.69,29.84 | 67.69,29.84 67.69,32.37 T3.1 | R17.2 68.29,29.25 67.69,29.84
  Bottom 0.254: PIC.59 69.83,24.23 v67.69,22.1
OUT_RELAY4  (via drill 0.6)
  Top 0.254: v69.22,21.72 69.22,24.77 70.61,26.16 70.61,29.21 72.01,30.61 72.01,35.2 T4.1 74.19,35.63 R16.2
  Bottom 0.254: PIC.60 70.33,23.98 69.34,22.99 69.34,21.84 v69.22,21.72
SRY0V.2
  Top 1.27: PRY0V.4.1 69.51,36.83 T4.3
SRY0V.3
  Top 1.27: PRY0V.3.1 64.43,34.8 T3.3
WIFI_IN_DEBUG_TX  (via drill 0.6)
  Top 0.254: v82.55,24.89 82.55,26.54 85.09,29.08 87.12,29.08 88.33,30.29 WIFIMOD.27 88.33,30.41 v88.9,29.84
  Bottom 0.254: PIC.2 75.39,23.57 76.33,24.51 82.17,24.51 v82.55,24.89 | v88.9,29.84 98.3,29.84 WTX.1
WIFI_IN_INT_INV  (via drill 0.6)
  Top 0.254: WIFIMOD.33 80.71,30.42 72.26,21.97 v72.26,20.45
  Top 0.406: R1.2 80.71,33.69 WIFIMOD.33
  Bottom 0.254: PIC.8 72.39,20.57 v72.26,20.45
WIFI_IN_SDI  (via drill 0.6)
  Top 0.254: WIFIMOD.32 81.98,27.88 v76.71,22.61
  Bottom 0.254: 76.2,22.1 v76.71,22.61 76.17,22.07 PIC.5
WIFI_OUT_CS_INV  (via drill 0.6)
  Top 0.254: WIFIMOD.23 93.41,30.16 93.09,29.84 90.93,29.84 89.53,28.45 86.11,28.45 v84.07,26.42
  Bottom 0.254: v84.07,26.42 80.39,26.42 78.99,25.02 75.18,25.02 PIC.1
WIFI_OUT_DEBUG_RX
  Top 0.254: 89.53,31.59 WRX.1 89.53,35.47 R12.1
  Top 0.406: 89.53,31.59 WIFIMOD.26
WIFI_OUT_HIBERNATE  (via drill 0.6)
  Top 0.254: WIFIMOD.20 97.22,29.66 96.27,28.7 90.81,28.7 86.87,24.77 v84.84,24.77
  Bottom 0.254: PIC.3 75.64,23.06 76.45,23.88 83.95,23.88 v84.84,24.77
WIFI_OUT_RESETINV  (via drill 0.6)
  Top 0.254: WIFIMOD.7 84.52,10.86 v81.66,13.72
  Bottom 0.254: v81.66,13.72 79.5,13.72 76.45,16.76 76.45,18.29 76.17,18.57 PIC.12
WIFI_OUT_SCK  (via drill 0.6)
  Top 0.254: WIFIMOD.34 79.44,30.42 78.74,29.72 77.98,29.72 72.14,23.88 v72.14,23.37
  Bottom 0.254: PIC.4 72.8,22.58 v72.14,23.37
WIFI_OUT_SDO  (via drill 0.6)
  Top 0.254: WIFIMOD.35 78.17,30.93 70.23,22.99 70.23,22.1 v70.74,21.59
  Bottom 0.254: v70.74,21.59 71.75,21.59 71.78,21.57 PIC.6
WIFI_OUT_WPINV  (via drill 0.6)
  Top 0.254: WIFIMOD.16 95.95,10.98 94.87,12.06 85.34,12.06 v81.53,15.88
  Bottom 0.254: v81.53,15.88 78.11,15.88 76.96,17.02 76.96,18.8 76.68,19.07 PIC.11

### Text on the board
tPlace: WISTEER V2 / mmm@devbooster.com | <L | <N
bPlace: WISTEER V2 / mmm@devbooster.com | <L | <N
bNames: Copyright (C) 2014-2015 / Marc Mirti Mancinelli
